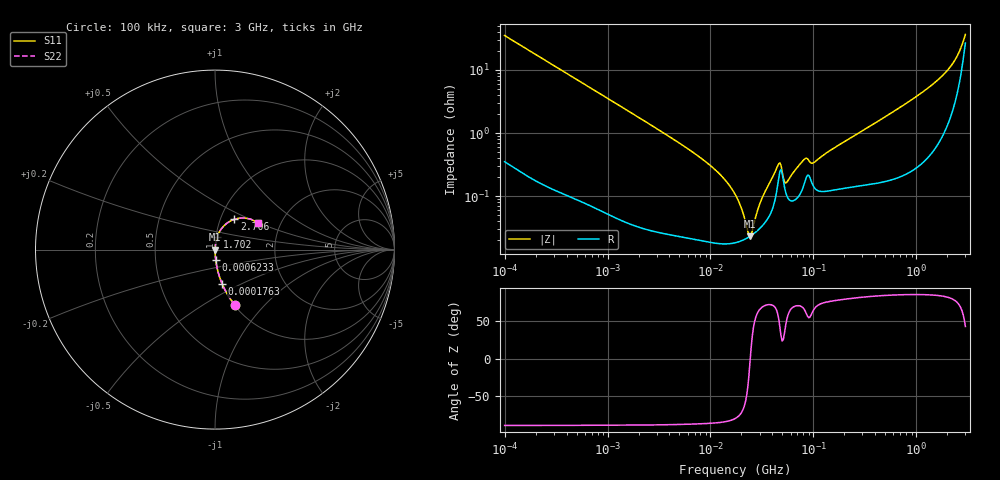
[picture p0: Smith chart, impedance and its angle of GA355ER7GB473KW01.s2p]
!Murata Part Number: GA355ER7GB473KW01
!These Parameters are Measured in Series Mode Connection
!Data Generated on Jun 19, 2026
!  o--ll--o
!Port1  Port2
!  o------o
!Operation Temp=25[degC], DC Bias Voltage=0[V]
!Freq. Start=100[kHz] Stop=3[GHz] 401[Steps]
# Hz S RI R 50
!Freq.(Hz) S11(Real) S11(Imag) S21(Real) S21(Imag) S12(Real) S12(Imag) S22(Real) S22(Imag)
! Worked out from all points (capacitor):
!   401 points, 100 kHz to 3 GHz, reference 50 ohm
!   read as one part in series: C = 45.3 nF near 105.3 kHz
!   lowest |Z| = 23.2 mohm at 24.21 MHz (marker M1)
!   series resonance near 24.37 MHz, so ESL is about 940 pH
!   S11 on the Smith chart (normalised r, x): 100 kHz: 1.01, -0.70; 176.3 kHz: 1.00, -0.40; 623.3 kHz: 1.00, -0.11; 1.702 GHz: 1.02, +0.15; 2.706 GHz: 1.17, +0.41; 3 GHz: 1.53, +0.50
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100000  0.1122 -0.3106  0.8878 0.3106  0.8878 0.3106  0.1122 -0.3106
176296  0.0401 -0.1914  0.9599 0.1914  0.9599 0.1914  0.0401 -0.1914
562235  0.00476 -0.0627  0.9952 0.0627  0.9952 0.0627  0.00476 -0.0627
623288  0.00397 -0.0566  0.996 0.0566  0.996 0.0566  0.00397 -0.0566
3161081  0.000389 -0.0112  0.9996 0.0112  0.9996 0.0112  0.000389 -0.0112
1.034438e7  0.000191 -0.00291  0.9998 0.00291  0.9998 0.00291  0.000191 -0.00291
1.409348e7  0.000178 -0.00175  0.9998 0.00175  0.9998 0.00175  0.000178 -0.00175
1.77727e7  0.000185 -0.000984  0.9998 0.000984  0.9998 0.000984  0.000185 -0.000984
2.421403e7  0.000231 -1.97e-05  0.9998 1.97e-05  0.9998 1.97e-05  0.000231 -1.97e-05
2.549486e7  0.000245 0.000142  0.9998 -0.000142  0.9998 -0.000142  0.000245 0.000142
3.13325e7  0.000329 0.000822  0.9997 -0.000822  0.9997 -0.000822  0.000329 0.000822
4.494634e7  0.00149 0.00261  0.9985 -0.00261  0.9985 -0.00261  0.00149 0.00261
4.732384e7  0.0025 0.00224  0.9975 -0.00224  0.9975 -0.00224  0.0025 0.00224
5.246276e7  0.00138 0.000954  0.9986 -0.000954  0.9986 -0.000954  0.00138 0.000954
5.523785e7  0.00101 0.00132  0.999 -0.00132  0.999 -0.00132  0.00101 0.00132
8.130716e7  0.00155 0.00348  0.9984 -0.00348  0.9984 -0.00348  0.00155 0.00348
9.738194e7  0.00159 0.00292  0.9984 -0.00292  0.9984 -0.00292  0.00159 0.00292
5.475153e8  0.00216 0.0198  0.9978 -0.0198  0.9978 -0.0198  0.00216 0.0198
1.701687e9  0.0129 0.0728  0.9871 -0.0728  0.9871 -0.0728  0.0129 0.0728
2.201951e9  0.0324 0.1115  0.9676 -0.1115  0.9676 -0.1115  0.0324 0.1115
2.706139e9  0.1086 0.169  0.8914 -0.169  0.8914 -0.169  0.1086 0.169
3e9  0.24 0.1495  0.76 -0.1495  0.76 -0.1495  0.24 0.1495
